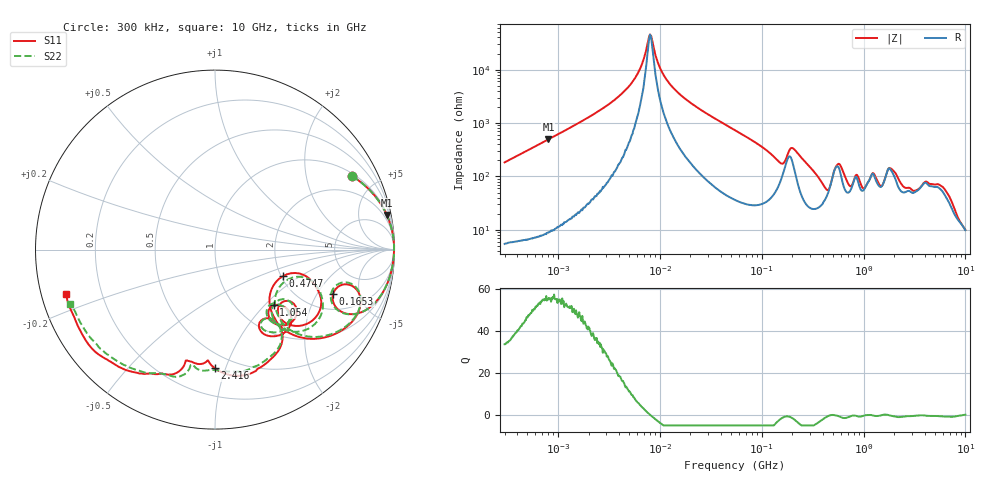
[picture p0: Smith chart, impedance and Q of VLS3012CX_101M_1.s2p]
! S-Parameter Data Generated by TDK Corporation
! Copyright(C) 2019 TDK Corporation.
! All Rights Reserved.
! TDK P/N: VLS3012CX-101M-1 (Inductor)
! Property: L=100uH at 1MHz
! Size(LxWxT): 3x3x1.2mm
! Model Type: s2p (Touchstone File Format Version 1.0)
! Frequency: DC=Yes Start=0.3MHz Stop=10000MHz 802points Log-sweep
! Model Generated on Sep. 23, 2019
! Port Assignments:
!  1 ---@@@--- 2
! Applicable Conditions:
!  Temperature = 25 degC
!  DC Bias Current = 0 A
!  Small Signal Operation
! Terms and conditions regarding TDK Simulation Models
! (1)This simulation model is being provided solely for informational purposes. Please refer to the specifications of the products in terms of detailed characteristics of such products.
! (2)In no event shall TDK Corporation of any of its subsidiaries be liable for any loss or damage arising, directly or indirectly,
!  From any information contained in this simulation model, including, but not limited to loss or damages arising from any inaccuracies, omissions or errors in connection with such information.
! (3)Any and all copyrights on this simulation model are owned by TDK Corporation.
!  Duplication or redistribution of this simulation model without prior written permission from TDK Corporation is prohibited.
! (4)This simulation model is subject to any modification or change without any prior notice.
! (5)Neither TDK Corporation nor any of its subsidiaries shall make any warranty, express or implied,
!  Including but not limited to the correctness, implied warranties of merchantability and fitness for a particular purpose with respect to this simulation models.
! (6)The use of this simulation model shall be deemed to have consented to the terms and conditions hereof.
# Hz S MA R 50
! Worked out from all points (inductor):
!   801 points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, 300 kHz to 10 GHz, reference 50 ohm
!   read as one part in series: L = 96.9 uH near 318.3 kHz
!   highest Q = 55.2 at 808.6 kHz (marker M1), where L = 97.2 uH
!   self-resonance near 8.009 MHz
!   S11 on the Smith chart (normalised r, x): 300 kHz: 1.11, +3.67; 165.3 MHz: 2.86, -2.78; 474.7 MHz: 2.04, -0.72; 1.054 GHz: 1.46, -1.13; 2.416 GHz: 0.39, -0.92; 10 GHz: 0.07, -0.15
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300000  0.8668 28.2  0.4732 -60.1  0.473 -60.1  0.8666 28.2
808588  0.9764 11.4  0.1977 -77.6  0.1977 -77.6  0.9762 11.4
1713600  0.9938 5.2  0.09199 -83.5  0.09204 -83.5  0.9937 5.2
5044683  0.998 1.0  0.01991 -83.9  0.01987 -84.0  0.998 1.0
6556275  0.9979 0.3  0.008659 -76.1  0.00869 -76.6  0.998 0.3
7890546  0.9978 -0.2  0.002382 -21.3  0.002364 -22.4  0.9978 -0.2
9671944  0.9976 -0.7  0.007718 71.7  0.007718 71.7  0.9977 -0.7
1.49005e7  0.9969 -1.9  0.02627 82.1  0.02628 82.1  0.9969 -1.9
5.477226e7  0.9845 -9.2  0.1338 78.0  0.1338 78.0  0.9843 -9.2
1.323997e8  0.8627 -24.5  0.3651 54.0  0.3652 54.0  0.8599 -24.7
1.653189e8  0.7028 -20.5  0.3809 25.6  0.3809 25.6  0.6912 -20.3
1.968335e8  0.8377 -16.9  0.2417 36.3  0.2417 36.3  0.8319 -16.0
3.126428e8  0.7595 -40.7  0.5302 39.9  0.5302 39.9  0.762 -39.5
4.149731e8  0.4744 -48.0  0.666 13.6  0.6661 13.6  0.4921 -45.5
4.74732e8  0.4051 -21.5  0.5822 -6.5  0.5823 -6.5  0.4413 -21.9
5.497689e8  0.6182 -21.7  0.3749 -0.1  0.375 -0.1  0.6605 -25.0
6.490631e8  0.6333 -42.1  0.5167 16.0  0.5168 16.0  0.6327 -46.3
1.054047e9  0.4501 -43.3  0.5748 -17.3  0.5749 -17.3  0.4397 -43.1
1.767019e9  0.6427 -54.7  0.3588 -35.4  0.3588 -35.4  0.6422 -55.6
2.416286e9  0.6593 -90.2  0.4682 -27.5  0.4682 -27.6  0.6759 -87.4
6.091595e9  0.8317 -125.9  0.2626 -65.0  0.2627 -65.0  0.8127 -126.3
1e10  0.8675 -163.4  0.242 -88.5  0.2423 -88.6  0.8651 -159.5
